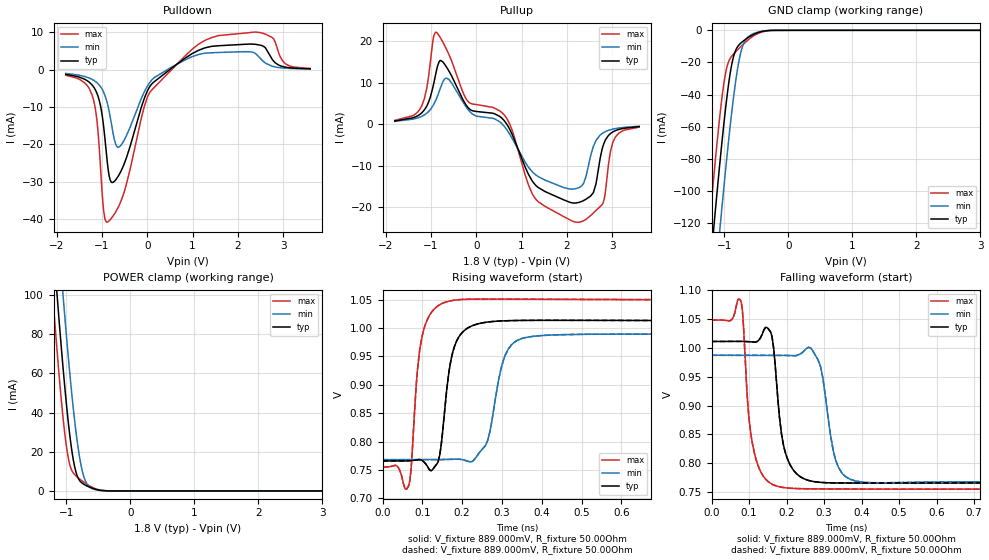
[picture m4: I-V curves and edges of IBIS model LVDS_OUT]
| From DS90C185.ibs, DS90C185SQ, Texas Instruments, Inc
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[Model]   LVDS_OUT
Model_type   Output
Vmeas = 0.900V
Rref = 50|100 Ohms Differential
|   typ   min   max
|   (nom)   (weak)   (fast)
C_comp   2.3129pF   2.3129pF   2.3129pF
[Voltage Range]   1.800V   1.710V   1.890V
[Temperature Range]   25.0   105.0   -40.0
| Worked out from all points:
|   slope of the pulldown table from 0 to 0.27 V, typ, clamps not added: 75.1 ohm
|   slope of the pullup table from 0 to 0.27 V, typ, clamps not added: 886 ohm
|   GND clamp passes 1 mA (typ) near -0.44 V on its own axis
|   POWER clamp passes 1 mA (typ) near -0.56 V on its own axis
|   falling waveform, V_fixture 889.000mV, R_fixture 50.00Ohm: 20-80 % time 27.8ps typ, 30.5ps min, 26.7ps max; typ from 1.01 V to 0.766 V
|   rising waveform, V_fixture 889.000mV, R_fixture 50.00Ohm: 20-80 % time 27.9ps typ, 36.4ps min, 23.5ps max; typ from 0.766 V to 1.01 V
|   rising waveform, V_fixture 889.000mV, R_fixture 50.00Ohm: 20-80 % time 27.9ps typ, 36.4ps min, 23.5ps max; typ from 0.766 V to 1.01 V
|   falling waveform, V_fixture 889.000mV, R_fixture 50.00Ohm: 20-80 % time 27.8ps typ, 30.5ps min, 26.7ps max; typ from 1.01 V to 0.766 V
[Pulldown]
|   Voltage   I(typ)   I(min)   I(max)
-1.8V     -1.276mA   -1.034mA   -1.502mA
-1.195V   -4.463mA   -2.769mA   -7.704mA
-1.114V   -6.247mA   -3.472mA   -13.33mA
-1.033V   -9.641mA   -4.562mA   -25.99mA
-963mV    -15.27mA   -6.069mA   -37.76mA
-887.4mV  -24.23mA   -8.756mA   -40.77mA
-801mV    -29.98mA   -13.85mA   -39.83mA
-612mV    -27.85mA   -20.6mA    -36.02mA
46.8mV    -4.675mA   -3.57mA    -6.253mA
1.127V    5.131mA    4.026mA    6.76mA
2.493V    6.534mA    3.021mA    9.886mA
3.595V    213.1uA    164.8uA    293.6uA
[GND Clamp]
|   Voltage   I(typ)   I(min)   I(max)
-1.8V     -420.3mA   -462.4mA   -389mA
-1.249V   -160.3mA   -203.2mA   -128.1mA
-1.228V   -150.6mA   -193.4mA   -118.4mA
-1.174V   -126.5mA   -169.1mA   -94.8mA
-1.141V   -112.4mA   -154.8mA   -81.09mA
-1.06V    -78.52mA   -119.7mA   -49.57mA
-968.4mV  -44.28mA   -82mA      -24.24mA
-865.8mV  -17.79mA   -44.63mA   -15.2mA
-736.2mV  -7.698mA   -12.74mA   -9.893mA
-590.4mV  -3.554mA   -2.937mA   -4.738mA
-244.8mV  -25.79uA   -23.77uA   -40.28uA
3.595V    0A         0A         0A
[Pullup]
|   Voltage   I(typ)   I(min)   I(max)
-1.8V     752.1uA    661.8uA    894.1uA
-1.201V   2.738mA    1.883mA    4.484mA
-871.2mV  13.28mA    6.376mA    21.99mA
-666mV    13.84mA    11.08mA    18.16mA
-180mV    3.93mA     3.467mA    5.403mA
667.8mV   58.42uA    -1.277mA   1.432mA
1.316V    -14.77mA   -12.24mA   -18.1mA
2.196V    -18.96mA   -15.51mA   -23.57mA
2.579V    -16.53mA   -5.486mA   -21.41mA
2.731V    -8.366mA   -2.674mA   -19.85mA
3.022V    -1.815mA   -1.176mA   -4.122mA
3.595V    -589.2uA   -521.8uA   -710.9uA
[POWER Clamp]
|   Voltage   I(typ)   I(min)   I(max)
-1.8V     403.8mA    442.1mA    375.8mA
-1.233V   138.2mA    177.5mA    108.9mA
-1.206V   126.4mA    165.5mA    97.18mA
-1.141V   98.66mA    137.3mA    70.17mA
-1.049V   62.2mA     99.15mA    36.75mA
-968.4mV  34.81mA    68.05mA    16.68mA
-882mV    14.28mA    39.32mA    8.775mA
-790.2mV  5.213mA    16.67mA    6.049mA
-703.8mV  2.981mA    5.218mA    3.982mA
-606.6mV  1.527mA    1.391mA    2.063mA
-352.8mV  30.38uA    29.93uA    39.08uA
3.595V    0A         0A         0A
[Ramp]
R_load = 50.00Ohm
|   typ   min   max
dV/dt_r   147.558mV/28.017ps  132.250mV/36.479ps  176.008mV/23.553ps
dV/dt_f   147.239mV/27.891ps  131.528mV/30.513ps  176.008mV/26.783ps
[Falling Waveform]
V_fixture = 889.000mV
V_fixture_min = 878.000mV
V_fixture_max = 890.000mV
R_fixture = 50.00Ohm
|   Time   V(typ)   V(min)   V(max)
0s        1.011V     987.2mV    1.048V
79.48ps   1.011V     987.1mV    1.079V
106.2ps   1.01V      987.2mV    844.2mV
157ps     1.028V     987.3mV    765.1mV
191.4ps   832.1mV    987mV      757.7mV
269.8ps   768.3mV    994.9mV    755.4mV
290.6ps   766.6mV    967.4mV    755.2mV
330.2ps   765.6mV    806.4mV    755.1mV
399.7ps   765.6mV    767.2mV    754.9mV
3.105ns   765.7mV    768mV      754.9mV
[Rising Waveform]
V_fixture = 889.000mV
V_fixture_min = 878.000mV
V_fixture_max = 890.000mV
R_fixture = 50.00Ohm
|   Time   V(typ)   V(min)   V(max)
0s        765.8mV    768mV      754.9mV
65.52ps   766mV      768mV      721.9mV
87.77ps   767.9mV    767.9mV    925.9mV
96.33ps   767.6mV    767.9mV    974.1mV
137.7ps   761.6mV    768.1mV    1.038V
180.6ps   967.2mV    768.9mV    1.049V
258.5ps   1.01V      792.8mV    1.051V
308.4ps   1.013V     952.3mV    1.051V
382.2ps   1.014V     985.7mV    1.051V
3.105ns   1.012V     988.4mV    1.048V
[Rising Waveform]
V_fixture = 889.000mV
V_fixture_min = 878.000mV
V_fixture_max = 890.000mV
R_fixture = 50.00Ohm
|   Time   V(typ)   V(min)   V(max)
0s        765.8mV    768mV      754.9mV
65.52ps   766mV      768mV      721.9mV
87.77ps   767.9mV    767.9mV    925.9mV
96.33ps   767.6mV    767.9mV    974.1mV
137.7ps   761.6mV    768.1mV    1.038V
180.6ps   967.2mV    768.9mV    1.049V
258.5ps   1.01V      792.8mV    1.051V
308.4ps   1.013V     952.3mV    1.051V
382.2ps   1.014V     985.7mV    1.051V
3.105ns   1.012V     988.4mV    1.048V
[Falling Waveform]
V_fixture = 889.000mV
V_fixture_min = 878.000mV
V_fixture_max = 890.000mV
R_fixture = 50.00Ohm
|   Time   V(typ)   V(min)   V(max)
0s        1.011V     987.2mV    1.048V
79.48ps   1.011V     987.1mV    1.079V
106.2ps   1.01V      987.2mV    844.2mV
157ps     1.028V     987.3mV    765.1mV
191.4ps   832.1mV    987mV      757.7mV
269.8ps   768.3mV    994.9mV    755.4mV
290.6ps   766.6mV    967.4mV    755.2mV
330.2ps   765.6mV    806.4mV    755.1mV
399.7ps   765.6mV    767.2mV    754.9mV
3.105ns   765.7mV    768mV      754.9mV
